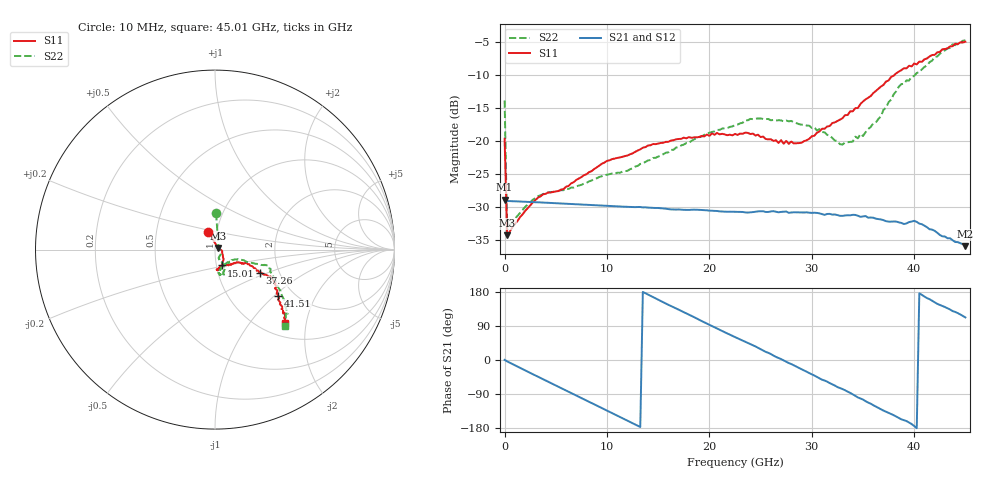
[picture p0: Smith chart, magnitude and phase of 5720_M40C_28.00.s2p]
! Device:  ADRF5720
! Description: 0.5dB LSB GaAs MMIC 6-bit Digital Attenuator
! Frequency:  0.000009 -  40 GHz
! Ports:
!	RF1	= Port 1
!	RF2	= Port 2
! Vdd:  3.3 Volt
! Vss:  -3.3 Volt
! Control:  0/3.3 Volt
! State:  28.00 dB attenuation
! Data:  The device was measured using G-S-G Probes on a matrix board.
!  Data was collected using an calibrated 4 port network analyzer.
!  The reference plane for this measurement is at the launchers.
! Note:  Analog Devices supplies this data as a sample of measured data
!  for this product.  Your particular data for this product may vary.
!  Data was taken at -40 degrees C.
!  Analog Devices reserves the right to change this data at anytime.
# GHZ S DB R 45.0
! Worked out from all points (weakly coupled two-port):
!   181 points, 10 MHz to 45.01 GHz, reference 45 ohm
!   highest |S21| = -28.85 dB at 10 MHz (marker M1); lowest = -35.9 dB at 45.01 GHz (marker M2)
!   lowest |S11| = -34.2 dB at 260 MHz (marker M3), VSWR 1.04, Z = 46.5 + j0.898 ohm
!   |S11| at or under -10 dB: start of sweep to 38.08 GHz
!   |S22| runs from -33.4 to -4.8 dB; largest |S21 - S12| = 0.00019
!   S11 on the Smith chart (normalised r, x): 10 MHz: 0.91, +0.18; 15.01 GHz: 1.06, -0.19; 37.26 GHz: 1.59, -0.45; 41.51 GHz: 1.67, -1.06; 45.01 GHz: 1.27, -1.52
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0.01  -19.64 110.8  -28.85 0.4  -28.88 0.3  -13.86 88.3
0.26  -34.22 29.7  -29.04 -3.7  -29.06 -3.7  -33.42 22.5
3.26  -28.54 -7.6  -29.24 -44.0  -29.27 -44.1  -28.31 -29.3
5.76  -27.26 -23.4  -29.43 -77.2  -29.45 -77.2  -27.41 -48.7
7.76  -25.14 -37.7  -29.59 -103.7  -29.61 -103.7  -26.41 -62.0
10.01  -22.98 -47.9  -29.78 -133.5  -29.80 -133.6  -25.07 -65.8
15.01  -20.37 -67.2  -30.10 159.3  -30.12 159.2  -22.33 -61.7
15.26  -20.27 -68.3  -30.13 155.7  -30.15 155.7  -22.18 -62.0
20.26  -18.82 -81.6  -30.51 89.4  -30.53 89.3  -18.61 -62.4
22.76  -19.06 -85.2  -30.70 57.3  -30.72 57.3  -17.50 -69.2
24.01  -18.92 -80.7  -30.76 42.0  -30.78 41.9  -16.63 -70.8
27.76  -20.40 -68.2  -30.83 -8.1  -30.86 -8.2  -17.00 -77.6
30.26  -19.18 -48.6  -30.82 -41.0  -30.85 -41.1  -17.91 -79.8
33.01  -16.54 -28.5  -31.29 -76.6  -31.31 -76.8  -20.51 -59.3
35.01  -14.01 -24.1  -31.37 -104.3  -31.40 -104.5  -19.22 -32.4
37.26  -10.99 -27.6  -32.09 -136.5  -32.10 -136.7  -14.94 -21.0
37.76  -10.28 -27.2  -32.16 -142.3  -32.19 -142.5  -13.73 -20.4
38.51  -9.49 -26.9  -32.27 -153.0  -32.30 -153.1  -11.76 -18.2
39.76  -8.70 -27.8  -32.15 -169.0  -32.15 -169.4  -10.27 -16.8
41.51  -7.20 -36.1  -33.31 160.4  -33.30 160.2  -8.06 -29.2
43.76  -5.65 -42.3  -34.97 129.1  -34.99 129.0  -5.35 -41.3
45.01  -4.97 -46.1  -35.87 112.3  -35.86 111.7  -4.78 -47.3
